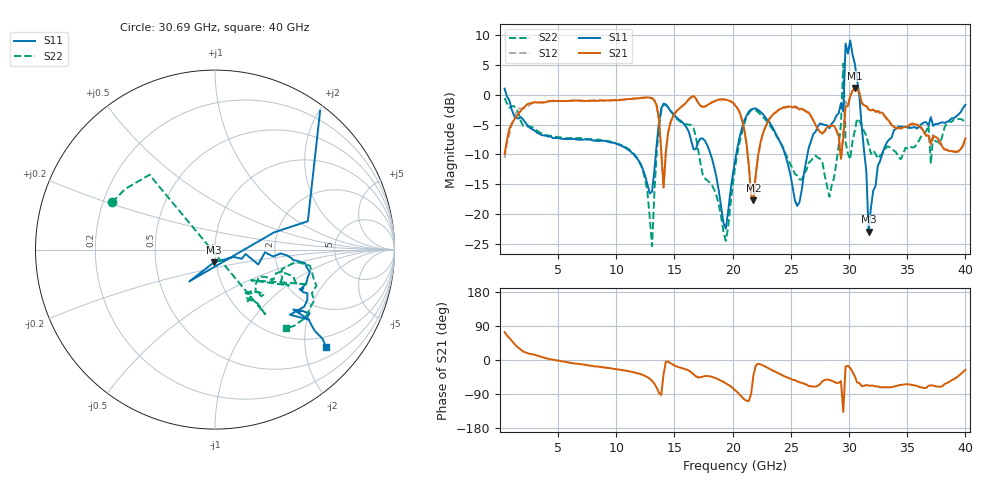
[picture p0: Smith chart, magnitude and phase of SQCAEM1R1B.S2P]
! Network Analyzer HP8722ES.07.66: Jul 25, 2000 Serial No. US39175408
! 26 Oct 2004  10:03:25
! Frequency  S11  S21  S12  S22
# HZ  S  DB R  50
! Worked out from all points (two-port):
!   201 points, 400 MHz to 40 GHz, reference 50 ohm
!   highest |S21| = 1.16 dB at 30.5 GHz (marker M1); lowest = -17.7 dB at 21.78 GHz (marker M2)
!   |S21| within 3 dB of the highest: 2.22 GHz to 13.47 GHz (11.25 GHz wide, 143 % of centre); 17.73 GHz to 20.24 GHz (2.51 GHz wide, 13.2 % of centre)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
!   lowest |S11| = -22.9 dB at 31.68 GHz (marker M3), VSWR 1.15, Z = 48.9 - j6.99 ohm
!   |S11| at or under -10 dB: 11.51 GHz to 13.39 GHz (1.887 GHz wide, 15.2 % of centre); 18.11 GHz to 20.3 GHz (2.193 GHz wide, 11.4 % of centre); 24.51 GHz to 26.43 GHz (1.921 GHz wide, 7.54 % of centre)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
!   |S22| runs from -25.4 to 5.2 dB; largest |S21 - S12| = 0.16
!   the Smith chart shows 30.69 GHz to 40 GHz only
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4e8  1.05 -17.1  -9.91 73.6  -10.61 78.5  -0.54 -9.9
1.588e9  -3.99 -62.7  -3.17 32.3  -2.29 33.5  -3.02 -51.2
7.132e9  -7.53 -97.6  -1.00 -11.9  -1.05 -12.7  -7.45 -108.3
1.3072e10  -16.22 -44.3  -0.57 -55.2  -0.58 -55.6  -25.36 98.5
1.3666e10  -4.62 -26.5  -4.13 -86.6  -4.21 -87.0  -5.29 -12.8
1.426e10  -1.61 -72.4  -9.54 -4.0  -9.42 -4.6  -1.68 -76.7
1.6636e10  -9.14 -114.2  -0.19 -37.5  -0.22 -37.8  -5.60 -151.3
1.9408e10  -22.43 -61.2  -0.82 -61.4  -0.82 -61.6  -24.47 110.1
2.02e10  -11.12 -12.8  -1.76 -79.5  -1.59 -79.6  -12.25 12.2
2.1784e10  -2.32 -62.6  -17.69 -40.0  -17.65 -37.2  -2.47 -77.8
2.5546e10  -18.62 -74.6  -2.13 -56.2  -2.20 -56.0  -13.51 128.7
2.6932e10  -6.56 -30.6  -4.27 -70.2  -4.35 -71.6  -10.46 23.8
2.9308e10  -1.40 -17.6  -10.72 -55.9  -10.64 -56.1  -4.82 19.6
2.9506e10  -2.78 12.3  -7.17 -136.9  -5.96 -119.4  5.22 44.3
2.9704e10  8.59 -7.8  -2.03 -17.1  -1.13 -7.9  -7.93 -65.0
2.9902e10  6.90 -62.2  -1.87 -15.1  -1.88 -15.2  -9.86 -0.2
3.01e10  9.11 -78.6  -0.22 -21.0  -0.35 -21.4  -10.80 7.2
3.0496e10  5.21 -103.0  1.16 -43.1  1.13 -43.9  -6.03 -11.1
3.0694e10  2.54 49.0  1.09 -59.2  0.98 -59.6  -3.99 155.4
3.1684e10  -22.92 -95.1  -2.46 -67.6  -2.44 -66.9  -8.39 -51.6
3.3466e10  -7.46 -6.0  -4.45 -71.8  -4.59 -72.5  -8.72 -45.3
4e10  -1.68 -41.3  -7.29 -26.0  -7.60 -25.9  -4.60 -48.2
